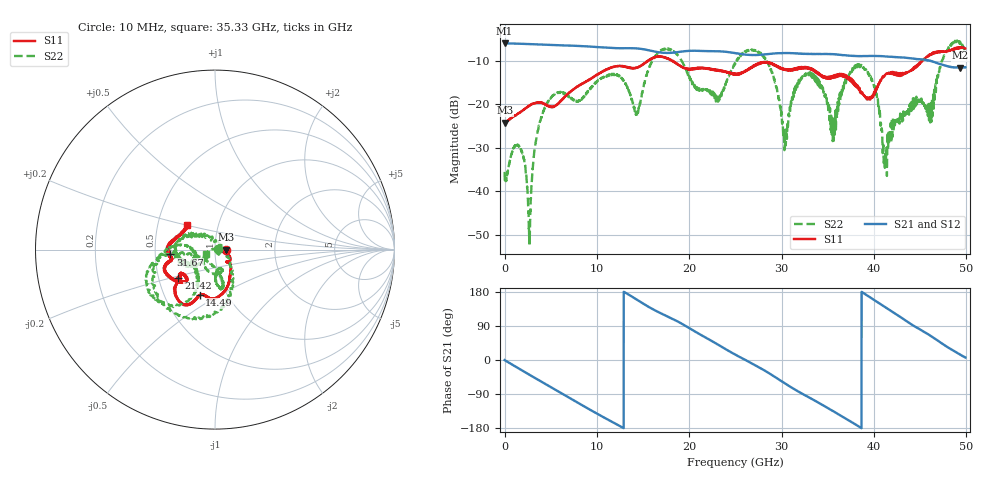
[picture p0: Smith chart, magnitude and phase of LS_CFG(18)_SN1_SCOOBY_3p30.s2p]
!Keysight Technologies,N5245B,MY58422026,A.13.80.08
!Date: Thursday, March 19, 2020 23:32:20
!Correction: S11(Full 2 Port(1,2))
!S21(Full 2 Port(1,2))
!S12(Full 2 Port(1,2))
!S22(Full 2 Port(1,2))
!S2P File: Measurements: S11, S21, S12, S22:
# Hz S DB R 50.0
!freq dBS11 angS11 dBS21 angS21 dBS12 angS12 dBS22 angS22
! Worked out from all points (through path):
!   4991 points, 10 MHz to 49.91 GHz, reference 50 ohm
!   highest |S21| = -5.99 dB at 10 MHz (marker M1); lowest = -11.6 dB at 49.35 GHz (marker M2)
!   group delay of S21, straight-line fit = 39.3 ps
!   lowest |S11| = -24.2 dB at 50 MHz (marker M3), VSWR 1.13, Z = 56.6 - j0.0402 ohm
!   |S11| at or under -10 dB: start of sweep to 15.57 GHz; 18.05984 GHz to 18.09128 GHz (31.44 MHz wide, 0.174 % of centre); 18.14 GHz to 45.24 GHz (27.1 GHz wide, 85.5 % of centre)
!   |S22| runs from -52.6 to -5.3 dB; largest |S21 - S12| = 0.0048
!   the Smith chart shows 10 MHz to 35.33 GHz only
!   S11 on the Smith chart (normalised r, x): 10 MHz: 1.13, -0.01; 14.49 GHz: 0.75, -0.41; 21.42 GHz: 0.63, -0.22; 31.67 GHz: 0.60, -0.03; 35.33 GHz: 0.70, +0.20
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1e7  -24.21 -3.3  -5.99 -0.3  -5.98 -0.3  -35.53 4.3
5e7  -24.22 -0.3  -5.99 -0.8  -5.99 -0.8  -37.59 -10.3
1.65e9  -21.91 -20.0  -6.09 -24.0  -6.09 -23.9  -29.84 -36.4
2.7e9  -20.30 -28.2  -6.18 -39.0  -6.17 -39.0  -52.59 85.5
4.42e9  -19.94 -45.1  -6.32 -63.4  -6.31 -63.4  -20.41 -134.1
8.33e9  -15.45 -60.7  -6.63 -118.3  -6.62 -118.2  -18.81 -81.7
1.204e10  -11.31 -90.1  -7.10 -168.4  -7.09 -168.4  -13.19 -80.6
1.449e10  -11.48 -108.6  -7.21 156.9  -7.20 157.0  -21.44 -144.4
1.665e10  -9.07 -120.6  -8.04 126.5  -8.02 126.6  -8.14 -162.0
2.142e10  -11.74 -142.0  -7.76 64.1  -7.76 64.2  -16.57 -147.1
2.496e10  -13.12 -140.8  -8.22 14.6  -8.21 14.7  -10.70 -174.3
2.827e10  -10.31 -156.4  -8.53 -29.3  -8.54 -29.2  -9.52 -84.0
3.038e10  -12.01 -167.5  -8.24 -61.9  -8.24 -61.8  -27.34 40.7
3.167e10  -12.03 -173.9  -8.33 -81.3  -8.34 -81.0  -15.85 153.2
3.328e10  -11.87 170.7  -8.44 -103.1  -8.44 -102.7  -13.12 -166.6
3.533e10  -13.63 139.4  -8.47 -131.2  -8.42 -130.9  -25.02 -154.8
3.851e10  -17.31 96.1  -8.93 -177.6  -8.91 -177.9  -11.11 -151.3
4.119e10  -13.32 35.1  -9.01 140.0  -9.03 139.8  -34.61 29.6
4.16e10  -12.74 33.0  -9.06 133.6  -9.08 133.5  -26.49 127.7
4.675e10  -7.91 -26.6  -10.47 53.9  -10.50 54.0  -14.89 -136.0
4.935e10  -6.94 -53.0  -11.57 14.1  -11.59 14.2  -5.70 -29.6
4.991e10  -7.19 -50.1  -11.49 6.5  -11.52 6.3  -7.83 -14.7
